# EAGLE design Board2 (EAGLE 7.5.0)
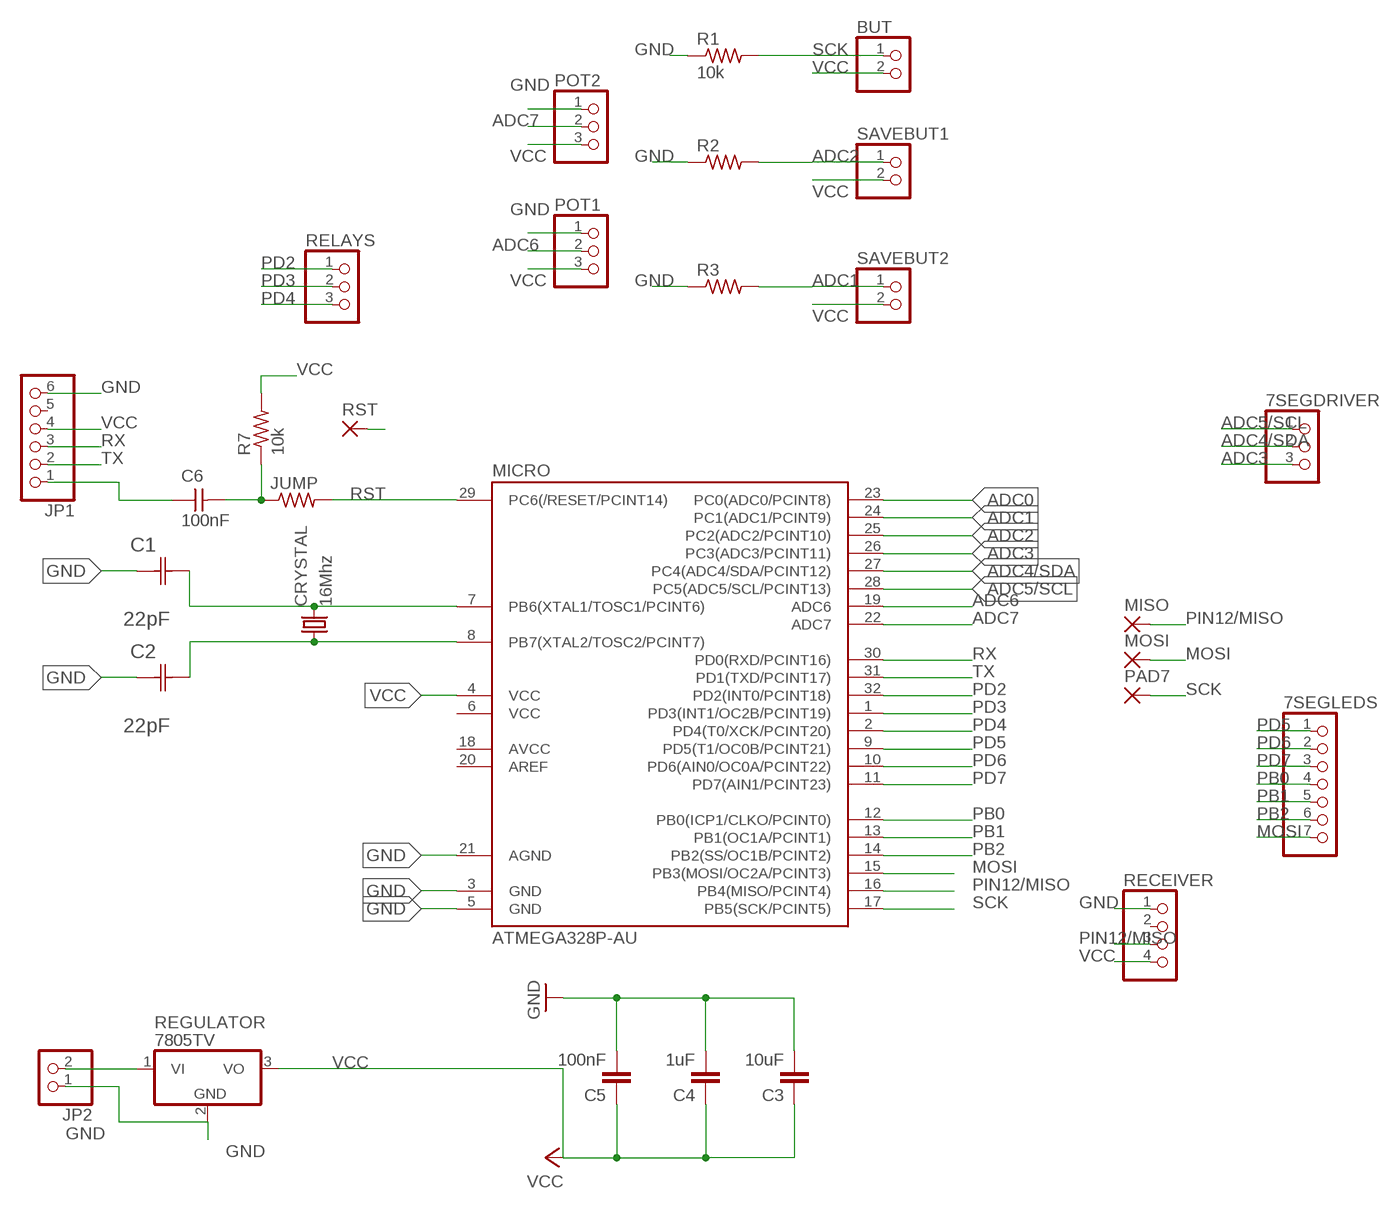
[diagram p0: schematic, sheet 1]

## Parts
7SEGDRIVER  PINHD-1X3  [1X03]
7SEGLEDS  PINHD-1X7  [1X07]
BUT  PINHD-1X2  [1X02]
C1  22pF  0612ZC225MAT2A  [CAPC3216X178N]
C2  22pF  0612ZC225MAT2A  [CAPC3216X178N]
C3  10uF  CAP1206  [1206]
C4  1uF  CAP1206  [1206]
C5  100nF  CAP1206  [1206]
C6  100nF  CAP-UNPOLARIZEDFAB  [C1206FAB]
CRYSTAL  16Mhz  CSM-7X-DU  [CSM-7X-DU]
JP1  PINHD-1X6  [1X06]
JP2  PINHD-1X2  [1X02]
JUMP  RES-US1206FAB  [R1206FAB]
MICRO  ATMEGA328P-AU  ATMEGA48/88/168-AU  [TQFP32-08]
MISO  1,6/0,8  [1,6/0,8]
MOSI  1,6/0,8  [1,6/0,8]
PAD7  1,6/0,8  [1,6/0,8]
POT1  PINHD-1X3  [1X03]
POT2  PINHD-1X3  [1X03]
R1  10k  RES-US1206FAB  [R1206FAB]
R2  RES-US1206FAB  [R1206FAB]
R3  RES-US1206FAB  [R1206FAB]
R7  10k  RES-US1206FAB  [R1206FAB]
RECEIVER  PINHD-1X4  [1X04]
REGULATOR  7805TV  [TO220V]
RELAYS  PINHD-1X3  [1X03]
RST  1,6/0,8  [1,6/0,8]
SAVEBUT1  PINHD-1X2  [1X02]
SAVEBUT2  PINHD-1X2  [1X02]

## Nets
ADC0: MICRO.23(PC0(ADC0/PCINT8))
ADC1: MICRO.24(PC1(ADC1/PCINT9)) R3.2 SAVEBUT2.1
ADC2: MICRO.25(PC2(ADC2/PCINT10)) R2.2 SAVEBUT1.1
ADC3: 7SEGDRIVER.3 MICRO.26(PC3(ADC3/PCINT11))
ADC4/SDA: 7SEGDRIVER.2 MICRO.27(PC4(ADC4/SDA/PCINT12))
ADC5/SCL: 7SEGDRIVER.1 MICRO.28(PC5(ADC5/SCL/PCINT13))
ADC6: MICRO.19(ADC6) POT1.2
ADC7: MICRO.22(ADC7) POT2.2
GND: C1.1(C1) C2.1(C1) C3.2 C4.2 C5.2 JP1.6 JP2.1 MICRO.3(GND) MICRO.5(GND) MICRO.21(AGND) POT1.1 POT2.1 R1.1 R2.1 R3.1 RECEIVER.1 REGULATOR.2(GND)
MOSI: 7SEGLEDS.7 MICRO.15(PB3(MOSI/OC2A/PCINT3)) MOSI.1(P)
N$1: JP2.2 REGULATOR.1(VI)
N$2: C1.2(C2) CRYSTAL.2 MICRO.7(PB6(XTAL1/TOSC1/PCINT6))
N$9: C2.2(C2) CRYSTAL.1 MICRO.8(PB7(XTAL2/TOSC2/PCINT7))
N$16: C6.1 JP1.1
PB0: 7SEGLEDS.4 MICRO.12(PB0(ICP1/CLKO/PCINT0))
PB1: 7SEGLEDS.5 MICRO.13(PB1(OC1A/PCINT1))
PB2: 7SEGLEDS.6 MICRO.14(PB2(SS/OC1B/PCINT2))
PD2: MICRO.32(PD2(INT0/PCINT18)) RELAYS.1
PD3: MICRO.1(PD3(INT1/OC2B/PCINT19)) RELAYS.2
PD4: MICRO.2(PD4(T0/XCK/PCINT20)) RELAYS.3
PD5: 7SEGLEDS.1 MICRO.9(PD5(T1/OC0B/PCINT21))
PD6: 7SEGLEDS.2 MICRO.10(PD6(AIN0/OC0A/PCINT22))
PD7: 7SEGLEDS.3 MICRO.11(PD7(AIN1/PCINT23))
PIN12/MISO: MICRO.16(PB4(MISO/PCINT4)) MISO.1(P) RECEIVER.3
RST: C6.2 JUMP.1 JUMP.2 MICRO.29(PC6(/RESET/PCINT14)) R7.1 RST.1(P)
RX: JP1.3 MICRO.30(PD0(RXD/PCINT16))
SCK: BUT.1 MICRO.17(PB5(SCK/PCINT5)) PAD7.1(P) R1.2
TX: JP1.2 MICRO.31(PD1(TXD/PCINT17))
VCC: BUT.2 C3.1 C4.1 C5.1 JP1.4 MICRO.4(VCC) POT1.3 POT2.3 R7.2 RECEIVER.4 REGULATOR.3(VO) SAVEBUT1.2 SAVEBUT2.2
Unconnected: JP1.5 MICRO.18(AVCC) MICRO.20(AREF) RECEIVER.2

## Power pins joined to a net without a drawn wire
VCC: MICRO.6(VCC)

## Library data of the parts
7SEGDRIVER POT1 POT2 RELAYS = pinhead:PINHD-1X3: PIN HEADER
7SEGLEDS = pinhead:PINHD-1X7: PIN HEADER
BUT JP2 SAVEBUT1 SAVEBUT2 = pinhead:PINHD-1X2: PIN HEADER
C1 C2 = AVX_By_element14_Batch_1:0612ZC225MAT2A: Capacitor 1206; MPN: 0612ZC225MAT2A; OC_FARNELL: -; OC_NEWARK: 12N3209; SUPPLIER: AVX; TOLERANCE: ±20%; VALUE: 2.2µF; VOLTAGERATING: 10V
C3-C5 = 01_SparkFun:CAP: Capacitor
C6 = fab:CAP-UNPOLARIZED
CRYSTAL = 01_FAB_Hello:CSM-7X-DU: SMD CRYSTAL; OC_FARNELL: unknown; OC_NEWARK: unknown
JP1 = pinhead:PINHD-1X6: PIN HEADER
JUMP R1-R3 R7 = fab:RES-US: Resistor (US Symbol)
MICRO = atmega8:ATMEGA48/88/168
MISO MOSI PAD7 RST = wirepad:1,6/0,8: THROUGH-HOLE PAD
RECEIVER = pinhead:PINHD-1X4: PIN HEADER
REGULATOR = linear:78*: Positive VOLTAGE REGULATOR Source: http://cache.national.com/ds/LM/LM78L05.pdf http://www.fairchildsemi.com/ds/LM/LM7805.pdf

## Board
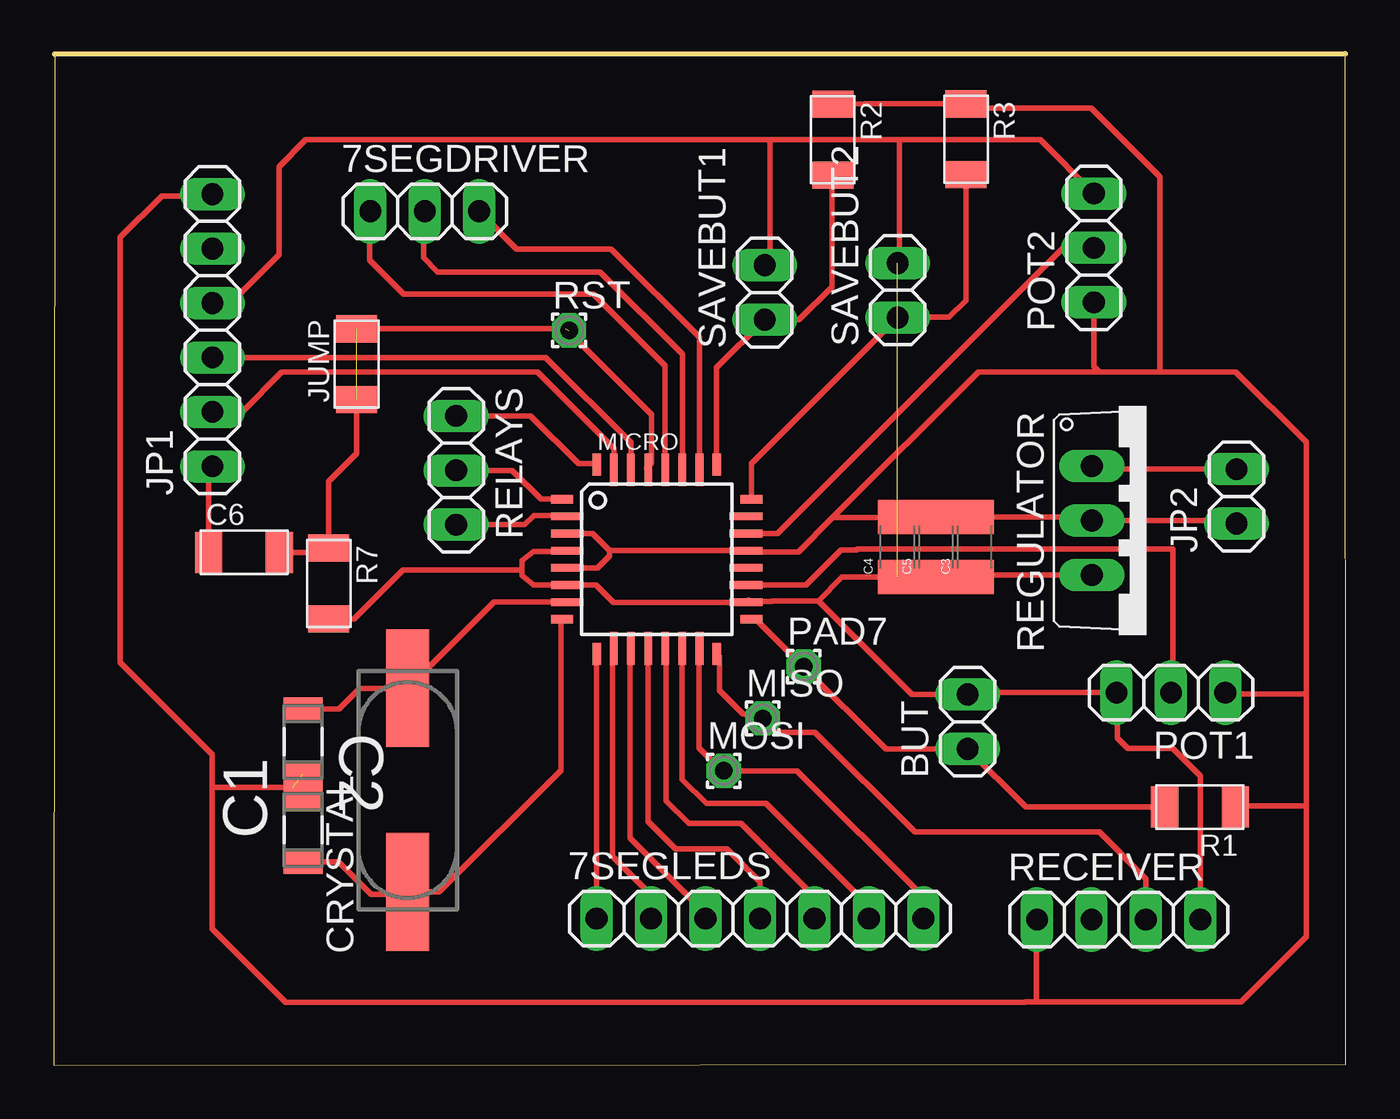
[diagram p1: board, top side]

Size 60.3 x 47.2 mm. Coordinates in mm from the lower left corner, seen from the top.
Outline: 0,0 60.3,0.03 60.27,47.2 0.05,47.17 0,0
Copper layers (1*16): Top 0.035mm / dielectric 1.5mm / Bottom 0.035mm
Design rules "default": minimum track width 10mil, minimum drill 24mil, track to track 8mil, track to pad 8mil, pad to pad 8mil, via to via 8mil, smd to smd 8mil, copper to edge 40mil, drill to drill 8mil, minimum pad ring 10mil, minimum via ring 8mil, stop-mask expansion 4mil, vias tented up to drill 0mil, thermal gap 10mil

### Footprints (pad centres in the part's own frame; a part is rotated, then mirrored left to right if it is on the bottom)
1X03 = drill 1.016 long: 1 -2.54,0; 2 0,0; 3 2.54,0
1X07 = drill 1.016 long: 1 -7.62,0; 2 -5.08,0; 3 -2.54,0; 4 0,0; 5 2.54,0; 6 5.08,0; 7 7.62,0
1X02 = drill 1.016 long: 1 -1.27,0; 2 1.27,0
CAPC3216X178N = smd 1.118 x 1.803: 1 -1.499,0; 2 1.499,0
1206 = smd 1.6 x 1.8: 1 -1.4,0; 2 1.4,0
C1206FAB = smd 1.27 x 1.905: 1 -1.651,0; 2 1.651,0
CSM-7X-DU = smd 5.5 x 2: 1 -4.75,0; 2 4.75,0
1X06 = drill 1.016 long: 1 -6.35,0; 2 -3.81,0; 3 -1.27,0; 4 1.27,0; 5 3.81,0; 6 6.35,0
R1206FAB = smd 1.27 x 1.905: 1 -1.651,0; 2 1.651,0
TQFP32-08 = smd 1.016 x 0.406: 1 -4.42,2.8; 8 -4.42,-2.8; 17 4.42,-2.8; 24 4.42,2.8 | smd 1.524 x 0.356: 2 -4.166,2; 3 -4.166,1.2; 4 -4.166,0.4; 5 -4.166,-0.4; 6 -4.166,-1.2; 7 -4.166,-2; 18 4.166,-2; 19 4.166,-1.2; 20 4.166,-0.4; 21 4.166,0.4; 22 4.166,1.2; 23 4.166,2 | smd 0.406 x 1.016: 9 -2.8,-4.42; 16 2.8,-4.42; 25 2.8,4.42; 32 -2.8,4.42 | smd 0.356 x 1.524: 10 -2,-4.166; 11 -1.2,-4.166; 12 -0.4,-4.166; 13 0.4,-4.166; 14 1.2,-4.166; 15 2,-4.166; 26 2,4.166; 27 1.2,4.166; 28 0.4,4.166; 29 -0.4,4.166; 30 -1.2,4.166; 31 -2,4.166
1,6/0,8 = drill 0.813 pad 1.6 octagon: 1 0,0
1X04 = drill 1.016 long: 1 -3.81,0; 2 -1.27,0; 3 1.27,0; 4 3.81,0
TO220V = drill 1.016 long: 1 -2.54,-2.54; 2 0,-2.54; 3 2.54,-2.54

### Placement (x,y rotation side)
7SEGDRIVER  17.32,39.84 0 top
7SEGLEDS  32.96,6.84 0 top
BUT  42.65,16.02 90 top
C1  11.64,15.09 90 top
C2  11.64,10.98 270 top
C3  42.98,24.17 90 top
C4  39.37,24.17 90 top
C5  41.18,24.17 90 top
C6  8.89,23.92 0 top
CRYSTAL  16.52,12.84 90 top
JP1  7.41,34.29 90 top
JP2  55.19,26.54 90 top
JUMP  14.14,32.71 90 top
MICRO  28.14,23.61 0 top
MISO  33.08,16.17 0 top
MOSI  31.27,13.73 0 top
PAD7  35,18.59 0 top
POT1  52.14,17.38 180 top
POT2  48.54,38.14 90 top
R1  53.49,12.04 180 top
R2  36.36,43.18 270 top
R3  42.57,43.2 270 top
R7  12.84,22.47 270 top
RECEIVER  49.7,6.79 0 top
REGULATOR  50.98,25.41 270 top
RELAYS  18.78,27.75 270 top
RST  24.05,34.28 0 top
SAVEBUT1  33.19,36.06 90 top
SAVEBUT2  39.38,36.16 90 top

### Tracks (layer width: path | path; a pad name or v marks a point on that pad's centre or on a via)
ADC1
  Top 0.254: MICRO.24 32.56,28.06 SAVEBUT2.1 39.39,34.9 41.78,34.9 42.57,35.68 R3.2
ADC2
  Top 0.254: MICRO.25 30.94,32.54 SAVEBUT1.1 34.78,34.79 36.31,36.31 36.31,41.48 R2.2
ADC3
  Top 0.254: 7SEGDRIVER.3 21.61,38.09 26.02,38.09 30.14,33.97 MICRO.26
ADC4/SDA
  Top 0.254: 7SEGDRIVER.2 17.25,39.78 17.25,37.68 17.92,37.01 25.5,37.01 29.34,33.18 MICRO.27
ADC5/SCL
  Top 0.254: 7SEGDRIVER.1 14.74,39.81 14.74,37.57 16.33,35.98 25.2,35.98 28.54,32.64 MICRO.28
ADC6
  Top 0.254: POT1.2 52.23,17.48 52.23,24.09 37.51,24.09 37.46,24.05 36.74,24.05 35.1,22.41 MICRO.19
ADC7
  Top 0.254: MICRO.22 33.77,24.8 47.1,38.14 POT2.2
GND  (1 unrouted)
  Top 0.254: JP2.1 55.05,25.41 REGULATOR.2 48.28,25.57 C3.2 C5.2 C4.2 39.34,25.54 36.35,25.54 | MICRO.3 25.15,24.81 25.94,24.01 | 25.94,24.01 25.94,23.76 25.37,23.2 23.98,23.2 MICRO.5 | 25.94,24.01 32.3,24.01 MICRO.21 32.37,23.94 34.75,23.94 36.35,25.54 | 58.44,17.32 58.44,29.07 55.17,32.34 51.61,32.34 | 51.61,32.34 48.79,32.34 | POT2.1 48.54,32.59 48.79,32.34 | POT1.1 54.74,17.32 58.44,17.32 | 45.85,2.95 45.36,2.95 45.33,2.93 10.83,2.93 7.39,6.37 7.39,12.68 7.39,12.96 | 45.85,2.95 55.41,2.95 58.44,5.98 58.44,12.09 | 58.44,12.09 58.44,17.32 | RECEIVER.1 45.85,6.75 45.85,2.95 | 36.35,25.54 43.14,32.34 48.79,32.34 | R1.1 55.18,12.09 58.44,12.09 | 51.61,32.34 51.61,41.45 48.42,44.64 42.78,44.64 R3.1 37.84,44.85 R2.1 | C2.1 11.16,12.96 7.39,12.96 | JP1.6 7.32,40.56 5.03,40.56 3.12,38.64 3.12,18.78 7.39,14.5 7.39,12.96
MOSI
  Top 0.254: MICRO.15 30.12,19.42 30.12,14.8 31.18,13.73 MOSI.1 34.69,13.73 40.6,7.83 40.6,6.86 7SEGLEDS.7
N$1
  Top 0.254: JP2.2 48.58,27.81 REGULATOR.1
N$2
  Top 0.254: C1.2 11.67,16.62 13.32,16.62 14.29,17.59 CRYSTAL.2 20.54,21.61 MICRO.7
N$9
  Top 0.254: MICRO.8 23.67,20.76 23.67,13.76 18,8.09 CRYSTAL.1 16.4,7.97 14.82,7.97 13.31,9.48 C2.2
N$16
  Top 0.254: 7.23,23.93 C6.1 7.24,27.77 JP1.1
PB0
  Top 0.254: MICRO.12 27.74,11.37 29.02,10.1 31.41,10.1 32.96,8.55 7SEGLEDS.4
PB1
  Top 0.254: MICRO.13 28.58,19.4 28.58,12.34 29.64,11.28 32.06,11.28 35.5,7.85 7SEGLEDS.5
PB2
  Top 0.254: MICRO.14 29.33,19.43 29.33,13.34 30.46,12.21 33.23,12.21 38.04,7.4 7SEGLEDS.6
PD2
  Top 0.254: RELAYS.1 22.27,30.29 24.48,28.08 25.29,28.08 MICRO.32
PD3
  Top 0.254: RELAYS.2 21.4,27.75 22.74,26.42 23.71,26.42 MICRO.1
PD4
  Top 0.254: RELAYS.3 21.99,25.21 22.42,25.65 23.93,25.65 MICRO.2
PD5
  Top 0.254: MICRO.9 7SEGLEDS.1
PD6
  Top 0.254: MICRO.10 26.09,19.39 26.09,9.74 27.88,7.95 7SEGLEDS.2
PD7
  Top 0.254: MICRO.11 26.9,19.41 26.9,10.61 30.42,7.09 7SEGLEDS.3
PIN12/MISO
  Top 0.254: MICRO.16 31.07,19.06 31.07,17.48 32.16,16.39 MISO.1 33.78,15.48 33.84,15.53 35.53,15.53 40.18,10.88 48.79,10.88 50.97,8.7 RECEIVER.3
RST  (2 unrouted)
  Top 0.254: MICRO.29 27.66,27.86 27.89,28.09 27.89,30.36 23.89,34.36 JUMP.2 | C6.2 12.64,23.92 R7.1 12.84,27.24 14.15,28.55 JUMP.1
RX
  Top 0.254: MICRO.30 26.94,29.05 22.96,33.02 JP1.3
SCK
  Top 0.254: MICRO.17 32.78,20.81 PAD7.1 38.83,14.75 BUT.1 45.36,12.04 R1.2
TX
  Top 0.254: MICRO.31 26.14,28.78 22.58,32.34 10.65,32.34 8.79,30.48 JP1.2
VCC  (1 unrouted)
  Top 0.254: 32.31,21.6 32.37,21.6 32.41,21.63 33.51,21.63 33.55,21.67 35.68,21.67 | 32.31,21.6 26.12,21.6 25.3,22.41 MICRO.6 22.39,22.41 21.85,22.84 21.85,23.1 | 21.85,23.1 21.85,23.55 22.39,23.98 23.94,23.98 MICRO.4 | REGULATOR.3 43.08,22.87 C3.1 C5.1 C4.1 36.78,22.77 35.68,21.67 | 21.85,23.1 16.3,23.1 14.03,20.82 R7.2 12.72,20.7 | 32.43,21.71 32.31,21.6 | BUT.2 42.74,17.38 POT1.3 49.63,17.35 49.63,15.26 50.11,14.78 52.23,14.78 53.51,13.5 RECEIVER.4 | 41.74,17.29 BUT.2 | 35.68,21.67 40.05,17.29 BUT.2 | POT2.3 46.03,43.18 39.45,43.18 | 39.45,43.18 33.43,43.18 | 33.43,43.18 11.77,43.18 10.51,41.92 10.51,37.81 8.27,35.56 JP1.4 | SAVEBUT1.2 33.43,37.57 33.43,43.18 | SAVEBUT2.2 39.45,37.5 39.45,43.18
